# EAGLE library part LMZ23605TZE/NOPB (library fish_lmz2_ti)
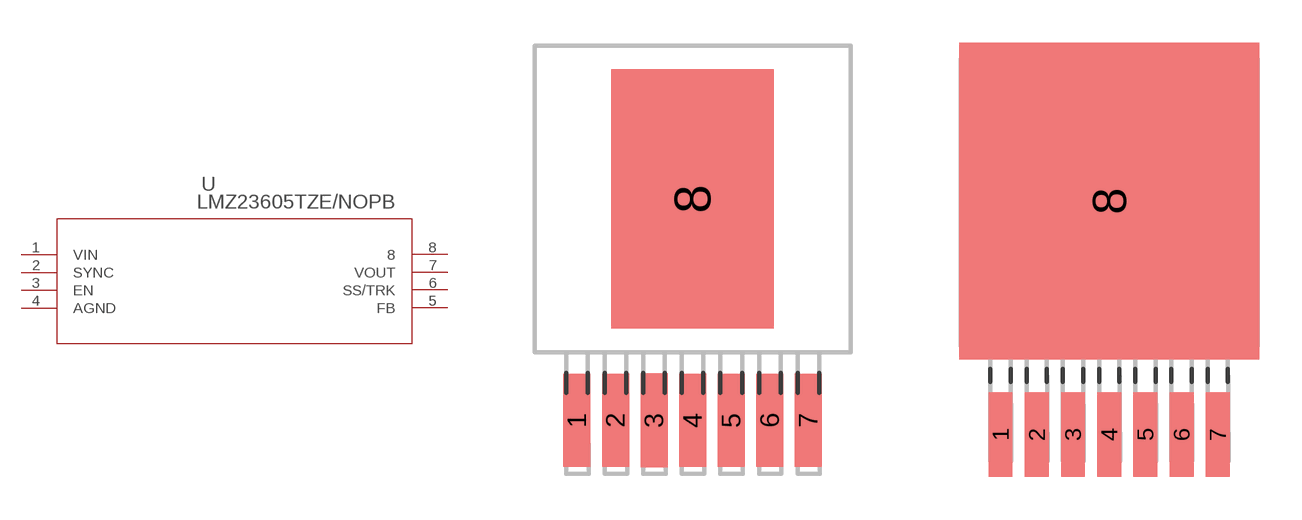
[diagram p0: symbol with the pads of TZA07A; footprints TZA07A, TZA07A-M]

Designator prefix U

## LMZ23605TZE/NOPB (MANUFACTURER_PART_NUMBER: LMZ23605TZENOPB; VENDOR: Texas Instruments)  [TZA07A]
1  VIN  in
2  SYNC  in
3  EN  in
4  AGND  pwr
5  FB  in
6  SS/TRK
7  VOUT  out
8  8  pas

## LMZ23605TZE/NOPBTZA07A-M (MANUFACTURER_PART_NUMBER: LMZ23605TZENOPB; VENDOR: Texas Instruments)  [TZA07A-M]
Pads as for TZA07A

## LMZ23605TZE/NOPBTZA07A-L (MANUFACTURER_PART_NUMBER: LMZ23605TZENOPB; VENDOR: Texas Instruments)  [TZA07A-L]
Pads as for TZA07A

## LMZ23605TZE/NOPBTZA07A-THERMAL  [TZA07A_THERMAL]
1  VIN  in
2  SYNC  in
3  EN  in
4  AGND  pwr
5  FB  in
6  SS/TRK
7  VOUT  out
8  8  pas
P$1  8  pas
P$2  8  pas
P$3  8  pas
P$4  8  pas
P$5  8  pas
P$6  8  pas
P$7  8  pas
P$8  8  pas
P$9  8  pas
P$10  8  pas
P$11  8  pas
P$12  8  pas
P$13  8  pas
P$14  8  pas
P$15  8  pas
P$16  8  pas
P$17  8  pas
P$18  8  pas
P$19  8  pas
P$20  8  pas
P$21  8  pas
P$22  8  pas
P$23  8  pas
P$24  8  pas
P$25  8  pas
P$26  8  pas
P$27  8  pas
P$28  8  pas
P$29  8  pas
P$30  8  pas
P$31  8  pas
P$32  8  pas
P$33  8  pas
P$34  8  pas
P$35  8  pas
P$36  8  pas
P$37  8  pas
P$38  8  pas
P$39  8  pas
P$40  8  pas
P$41  8  pas
P$42  8  pas
P$43  8  pas
P$44  8  pas
P$45  8  pas
P$46  8  pas
P$47  8  pas
P$48  8  pas
P$49  8  pas
P$50  8  pas
P$51  8  pas
P$52  8  pas
P$53  8  pas
P$54  8  pas

## Footprint TZA07A (pad centres in mm)
smd 0.89 x 3.06: 1 -3.81,-7.305; 2 -2.54,-7.305; 4 0,-7.305; 5 1.27,-7.305; 6 2.54,-7.305; 7 3.81,-7.305
smd 0.89 x 3.09: 3 -1.27,-7.305
smd 5.35 x 8.54: 8 0,0

## Footprint TZA07A-M (pad centres in mm)
smd 0.838 x 2.972: 1 -3.81,-8.141; 2 -2.54,-8.141; 3 -1.27,-8.141; 4 0,-8.141; 5 1.27,-8.141; 6 2.54,-8.141; 7 3.81,-8.141
smd 10.516 x 11.125: 8 0,0.051

## Footprint TZA07A-L (pad centres in mm)
smd 0.737 x 2.362: 1 -3.81,-8.039; 2 -2.54,-8.039; 3 -1.27,-8.039; 4 0,-8.039; 5 1.27,-8.039; 6 2.54,-8.039; 7 3.81,-8.039
smd 10.414 x 10.516: 8 0,-0.051

## Footprint TZA07A_THERMAL (pad centres in mm)
smd 0.89 x 3.06: 1 -3.81,-7.305; 2 -2.54,-7.305; 4 0,-7.305; 5 1.27,-7.305; 6 2.54,-7.305; 7 3.81,-7.305
smd 0.89 x 3.09: 3 -1.27,-7.305
smd 5.512 x 8.661: 8 0,0
drill 0.254 pad 0.406: P$1 -2.464,3.81; P$2 -1.473,3.81; P$3 -0.483,3.81; P$4 0.508,3.81; P$5 1.499,3.81; P$6 2.489,3.81; P$7 -2.464,2.819; P$8 -1.473,2.819; P$9 -0.483,2.819; P$10 0.508,2.819; P$11 1.499,2.819; P$12 2.489,2.819; P$13 -2.464,1.829; P$14 -1.473,1.829; P$15 -0.483,1.829; P$16 0.508,1.829; P$17 1.499,1.829; P$18 2.489,1.829; P$19 -2.464,0.838; P$20 -1.473,0.838; P$21 -0.483,0.838; P$22 0.508,0.838; P$23 1.499,0.838; P$24 2.489,0.838; P$25 -2.464,-0.152; P$26 -1.473,-0.152; P$27 -0.483,-0.152; P$28 0.508,-0.152; P$29 1.499,-0.152; P$30 2.489,-0.152; P$31 -2.464,-1.143; P$32 -1.473,-1.143; P$33 -0.483,-1.143; P$34 0.508,-1.143; P$35 1.499,-1.143; P$36 2.489,-1.143; P$37 -2.464,-2.134; P$38 -1.473,-2.134; P$39 -0.483,-2.134; P$40 0.508,-2.134; P$41 1.499,-2.134; P$42 2.489,-2.134; P$43 -2.464,-3.124; P$44 -1.473,-3.124; P$45 -0.483,-3.124; P$46 0.508,-3.124; P$47 1.499,-3.124; P$48 2.489,-3.124; P$49 -2.464,-4.115; P$50 -1.473,-4.115; P$51 -0.483,-4.115; P$52 0.508,-4.115; P$53 1.499,-4.115; P$54 2.489,-4.115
